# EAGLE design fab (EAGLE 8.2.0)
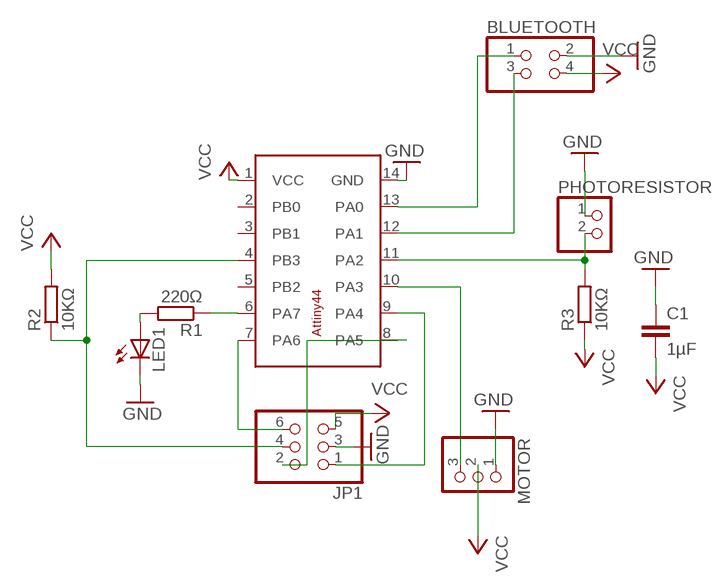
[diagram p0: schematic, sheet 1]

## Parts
BLUETOOTH  PINHD-2X2  [2X02]
C1  1µF  C-EUC1206  [C1206]
JP1  PINHD-2X3  [2X03]
LED1  LEDCHIPLED_1206  [CHIPLED_1206]
MOTOR  PINHD-1X3  [1X03]
PHOTORESISTOR  PINHD-1X2  [1X02]
R1  220Ω  R-EU_R1206  [R1206]
R2  10KΩ  R-EU_R1206  [R1206]
R3  10KΩ  R-EU_R1206  [R1206]
U$1  ATTINY44-SO14  [SO14]

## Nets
GND: BLUETOOTH.2 C1.1 JP1.3 LED1.C MOTOR.1 PHOTORESISTOR.1 U$1.14(GND)
MISO: JP1.2 U$1.8(PA5)
MOSI: JP1.6 U$1.7(PA6)
N$1: MOTOR.3 U$1.10(PA3)
N$5: LED1.A R1.2
N$6: R1.1 U$1.6(PA7)
N$8: PHOTORESISTOR.2 R3.2 U$1.11(PA2)
N$9: BLUETOOTH.3 U$1.12(PA1)
N$10: BLUETOOTH.1 U$1.13(PA0)
RESET: JP1.4 R2.1 U$1.4(PB3)
SCK: JP1.1 U$1.9(PA4)
VCC: BLUETOOTH.4 C1.2 JP1.5 MOTOR.2 R2.2 R3.1 U$1.1(VCC)
Unconnected: U$1.2(PB0) U$1.3(PB1) U$1.5(PB2)

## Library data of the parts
BLUETOOTH = pinhead:PINHD-2X2: PIN HEADER
C1 = rcl:C-EU: CAPACITOR, European symbol
JP1 = pinhead:PINHD-2X3: PIN HEADER
LED1 = led:LED: LED
MOTOR = pinhead:PINHD-1X3: PIN HEADER
PHOTORESISTOR = pinhead:PINHD-1X2: PIN HEADER
R1-R3 = resistor:R-EU_: RESISTOR, European symbol
U$1 = atmel-new:ATTINY44-SO14

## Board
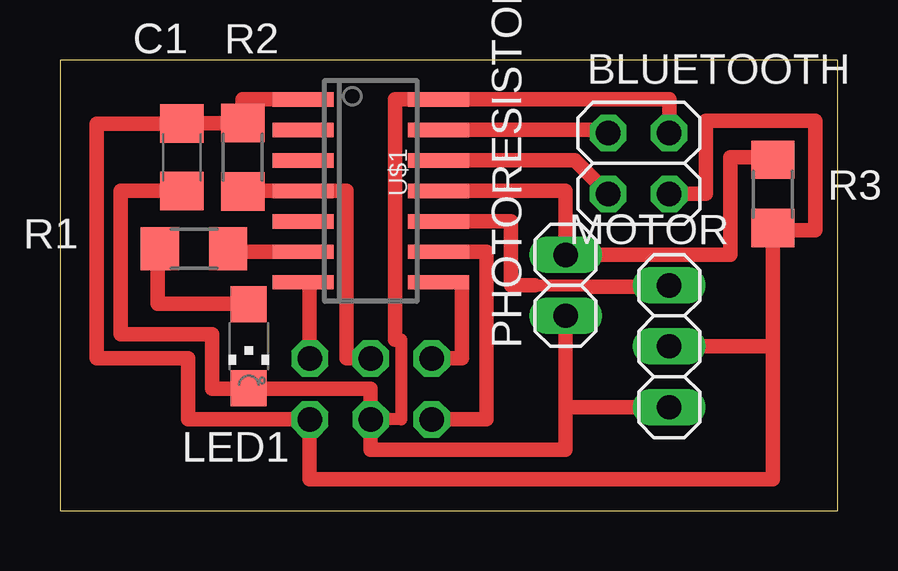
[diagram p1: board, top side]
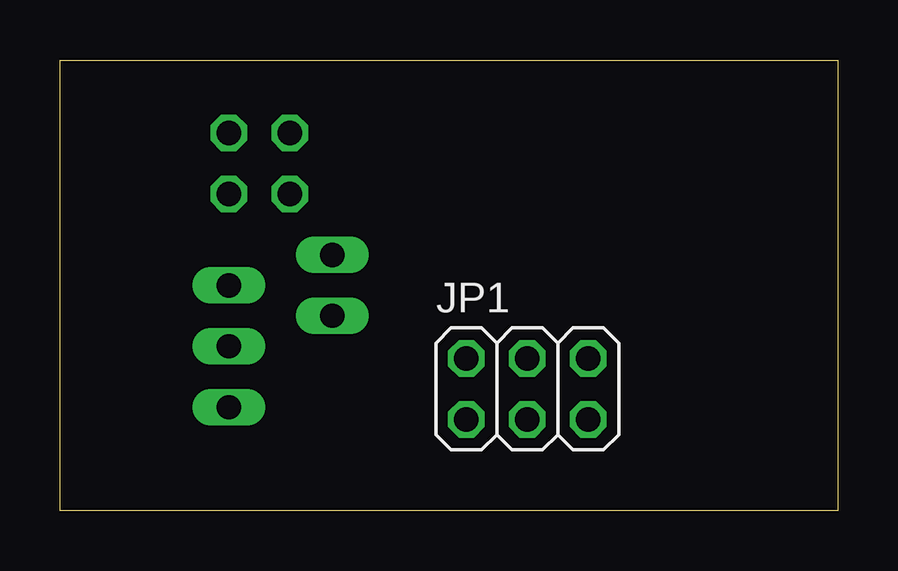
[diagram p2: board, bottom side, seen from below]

Size 32.44 x 18.79 mm. Coordinates in mm from the lower left corner, seen from the top.
Outline: 0,0 32.44,0 32.44,18.79 0,18.79 0,0
Copper layers (1*16): Top 0.035mm / dielectric 1.5mm / Bottom 0.035mm
Design rules "default *": minimum track width 24mil, minimum drill 24mil, track to track 8mil, track to pad 8mil, pad to pad 8mil, via to via 8mil, smd to smd 8mil, copper to edge 40mil, drill to drill 8mil, minimum pad ring 10mil, minimum via ring 8mil, stop-mask expansion 4mil, vias tented up to drill 0mil, thermal gap 10mil

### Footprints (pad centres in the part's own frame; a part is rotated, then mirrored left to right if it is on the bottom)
2X02 = drill 1.016 octagon: 1 -1.27,-1.27; 2 -1.27,1.27; 3 1.27,-1.27; 4 1.27,1.27
C1206 = smd 1.6 x 1.8: 1 -1.4,0; 2 1.4,0
2X03 = drill 1.016 octagon: 1 -2.54,-1.27; 2 -2.54,1.27; 3 0,-1.27; 4 0,1.27; 5 2.54,-1.27; 6 2.54,1.27
CHIPLED_1206 = smd 1.5 x 1.5: A 0,-1.75; C 0,1.75
1X03 = drill 1.016 long: 1 -2.54,0; 2 0,0; 3 2.54,0
1X02 = drill 1.016 long: 1 -1.27,0; 2 1.27,0
R1206 = smd 1.6 x 1.803: 1 -1.422,0; 2 1.422,0
SO14 = smd 0.6 x 2.54: 1 -3.175,-2.822; 2 -1.905,-2.822; 3 -0.635,-2.822; 4 0.635,-2.822; 5 1.905,-2.822; 6 3.175,-2.822; 7 4.445,-2.822; 8 4.445,2.822; 9 3.175,2.822; 10 1.905,2.822; 11 0.635,2.822; 12 -0.635,2.822; 13 -1.905,2.822; 14 -3.175,2.822

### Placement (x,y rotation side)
BLUETOOTH  24.13,14.48 270 top
C1  5.08,14.73 90 top
JP1  12.95,5.08 0 bottom
LED1  7.87,6.86 180 top
MOTOR  25.4,6.86 90 top
PHOTORESISTOR  21.08,9.4 90 top
R1  5.59,10.92 180 top
R2  7.62,14.73 90 top
R3  29.72,13.21 90 top
U$1  12.95,13.97 270 top

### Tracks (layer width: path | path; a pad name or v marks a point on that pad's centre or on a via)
GND
  Top 0.508: 13.97,7.13 14.22,7.13 14.22,3.81 JP1.3
  Top 0.61: BLUETOOTH.2 25.4,17.14 U$1.14 13.97,17.14 13.97,7.13 | 21.08,4.32 21.08,2.54 12.95,2.54 JP1.3 12.95,5.08 7.87,5.08 | 21.08,4.32 PHOTORESISTOR.1 | 7.87,5.08 6.35,5.08 6.35,7.37 2.54,7.37 2.54,13.33 C1.1 | LED1.C 7.87,5.08 | 21.08,4.32 MOTOR.1
MISO
  Top 0.61: JP1.2 16.76,6.35 16.76,9.52 U$1.8
MOSI
  Top 0.61: U$1.7 10.41,9.52 JP1.6
N$1
  Top 0.508: 19.79,9.4 22.05,9.4 22.1,9.35
  Top 0.61: U$1.10 18.8,12.07 18.8,9.4 19.79,9.4 | 22.1,9.35 25.4,9.35 MOTOR.3
N$5
  Top 0.61: 3.81,10.92 R1.2 4.06,10.92 4.06,8.64 7.87,8.64 LED1.A
N$6
  Top 0.61: U$1.6 7.01,10.79 R1.1
N$8
  Top 0.61: R3.2 29.75,14.61 | U$1.11 21.08,13.34 PHOTORESISTOR.2 27.94,10.67 27.94,14.73 29.72,14.73 R3.2 | 29.72,14.61 R3.2
N$9
  Top 0.61: U$1.12 21.46,14.61 BLUETOOTH.3
N$10
  Top 0.61: U$1.13 22.86,15.88 BLUETOOTH.1
RESET
  Top 0.61: R2.1 7.62,13.34 U$1.4 11.94,13.34 11.94,6.35 JP1.4
SCK
  Top 0.61: U$1.9 17.78,10.79 17.78,3.81 JP1.1
VCC
  Top 0.61: R3.1 29.59,11.75 | 29.72,6.86 29.72,4.83 | 29.72,4.83 29.72,4.32 | R3.1 29.72,6.86 | 29.72,12.07 R3.1 | U$1.1 7.62,17.14 R2.2 5.08,16.15 C1.2 1.52,16.13 1.52,6.35 5.33,6.35 5.33,3.81 JP1.5 10.41,1.32 23.11,1.32 | BLUETOOTH.4 26.92,13.21 26.92,16.26 31.5,16.26 31.5,11.68 29.72,11.68 R3.1 | MOTOR.2 29.72,6.86 | 29.72,4.83 29.72,1.32 23.11,1.32 | 23.11,1.32 21.52,1.32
